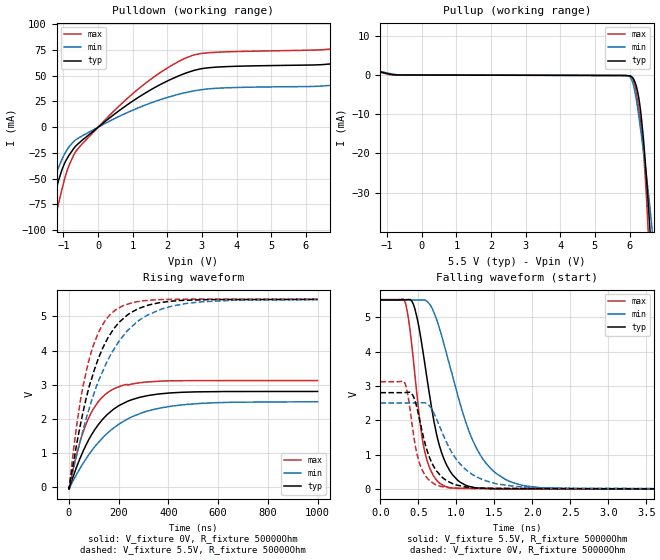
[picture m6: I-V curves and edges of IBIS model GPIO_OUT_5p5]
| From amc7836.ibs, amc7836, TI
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|   Model
[Model]   GPIO_OUT_5p5
Model_type   Output
Polarity   Non-Inverting
Vmeas = 2.75
Vref = 0
Cref = 1pF
Rref = 100000
|   typ   min   max
C_comp   2.855pF   2.622pF   2.914pF
[Voltage Range]   5.5   5.49   5.51
[Temperature Range]   27   125   -40
[Pullup Reference]   5.5   5.49   5.51
[Pulldown Reference]   0   0   0
[Power Clamp Reference]   5.5   5.49   5.51
[GND Clamp Reference]   0   0   0
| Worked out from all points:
|   slope of the pulldown table from 0 to 0.825 V, typ, clamps not added: 38.7 ohm
|   slope of the pullup table from 0 to 0.825 V, typ, clamps not added: 48 kohm
|   falling waveform, V_fixture 5.5V, R_fixture 50000Ohm: 20-80 % time 268ps typ, 471ps min, 181ps max; typ from 5.5 V to 0.008 V
|   rising waveform, V_fixture 0V, R_fixture 50000Ohm: 20-80 % time 143ns typ, 196ns min, 97.6ns max; typ from 0.004 V to 2.81 V
|   rising waveform, V_fixture 5.5V, R_fixture 50000Ohm: 20-80 % time 132ns typ, 177ns min, 93.2ns max; typ from 0.008 V to 5.5 V
|   falling waveform, V_fixture 0V, R_fixture 50000Ohm: 20-80 % time 236ps typ, 417ps min, 158ps max; typ from 2.81 V to 0.004 V
[Pulldown]
|   Voltage   I(typ)   I(min)   I(max)
-5.5V     -815mA     -579.5mA   -1.061A
-1.722V   -140.2mA   -96.71mA   -191.6mA
-1.359V   -81.74mA   -58.92mA   -111.9mA
-1.012V   -38.62mA   -28.98mA   -56.06mA
-632.5mV  -17.84mA   -11.99mA   -23mA
1.166V    28.92mA    18.78mA    37.11mA
2.767V    54.99mA    35.15mA    69.99mA
6.463V    60.57mA    39.89mA    74.99mA
8.129V    68.34mA    45.17mA    85.32mA
9.069V    77.47mA    50.99mA    97.72mA
10.18V    94.67mA    61.95mA    121.1mA
11V       112.3mA    74.03mA    145.2mA
[Pullup]
|   Voltage   I(typ)   I(min)   I(max)
-5.5V     9.928mA    9.651mA    11.85mA
-929.5mV  216.6uA    408.6uA    95.49uA
6.017V    -229.1uA   -533.7uA   -273.6uA
6.165V    -1.982mA   -4.705mA   -3.143mA
6.298V    -7.66mA    -12.35mA   -10.63mA
6.413V    -17.51mA   -20.18mA   -20.76mA
6.463V    -22.98mA   -23.73mA   -27.12mA
6.529V    -31.17mA   -28.79mA   -37.86mA
6.561V    -35.54mA   -31.49mA   -43.95mA
6.595V    -40.06mA   -34.28mA   -50.33mA
6.694V    -54.26mA   -43.07mA   -70.56mA
11V       -814.8mA   -580.7mA   -1.058A
[Ramp]
R_load = 50000
|   typ   min   max
dV/dt_r   1.6811/1.43476e-07   1.49998/1.96434e-07   1.87211/9.764e-08
dV/dt_f   3.29529/2.67942e-10   3.28767/4.70856e-10   3.30186/1.80999e-10
[Falling Waveform]
V_fixture = 5.5V
V_fixture_min = 5.49V
V_fixture_max = 5.51V
R_fixture = 50000Ohm
C_fixture = 0F
|   Time   V(typ)   V(min)   V(max)
0s        5.5V       5.49V      5.51V
329.1ps   5.505V     5.495V     5.416V
441.7ps   5.335V     5.497V     3.62V
561.9ps   3.991V     5.499V     1.348V
744ps     1.561V     4.912V     254.2mV
952.8ps   415.1mV    3.272V     36.64mV
1.312ns   33.4mV     1.005V     25.55mV
1.645ns   15.2mV     288.2mV    20.86mV
2.087ns   15.19mV    48.48mV    14.65mV
1us       7.874mV    10.86mV    6.893mV
[Rising Waveform]
V_fixture = 0V
V_fixture_min = 0V
V_fixture_max = 0V
R_fixture = 50000Ohm
C_fixture = 0F
|   Time   V(typ)   V(min)   V(max)
0s        3.959mV    4.903mV    3.844mV
576.4ps   -30.53mV   3.41mV     -54.48mV
21.56ns   407.6mV    256.6mV    684.5mV
43.6ns    830.4mV    539.8mV    1.31V
79.21ns   1.387V     947.3mV    2.028V
128.4ns   1.927V     1.391V     2.595V
187.6ns   2.326V     1.777V     2.906V
292.5ns   2.646V     2.177V     3.067V
415.5ns   2.765V     2.379V     3.118V
1us       2.806V     2.505V     3.124V
[Rising Waveform]
V_fixture = 5.5V
V_fixture_min = 5.49V
V_fixture_max = 5.51V
R_fixture = 50000Ohm
C_fixture = 0F
|   Time   V(typ)   V(min)   V(max)
0s        7.874mV    10.86mV    6.893mV
43.6ns    1.746V     1.302V     2.422V
79.21ns   2.89V      2.254V     3.686V
128.4ns   3.948V     3.267V     4.674V
187.6ns   4.706V     4.118V     5.189V
234.1ns   5.038V     4.577V     5.357V
292.5ns   5.265V     4.939V     5.451V
415.5ns   5.45V      5.305V     5.502V
669.7ns   5.496V     5.476V     5.509V
1us       5.5V       5.49V      5.51V
[Falling Waveform]
|Gnd
V_fixture = 0V
V_fixture_min = 0V
V_fixture_max = 0V
R_fixture = 50000Ohm
C_fixture = 0F
|   Time   V(typ)   V(min)   V(max)
0s        2.806V     2.505V     3.124V
319.4ps   2.809V     2.505V     3.101V
412.9ps   2.786V     2.505V     1.971V
509.4ps   2.102V     2.511V     804mV
612.2ps   1.148V     2.485V     337.8mV
711.4ps   630.3mV    2.182V     154.5mV
961.8ps   154mV      994.9mV    37mV
1.267ns   38.86mV    357.8mV    22.39mV
2.619ns   18.54mV    28.99mV    8.69mV
1us       3.959mV    4.903mV    3.844mV
